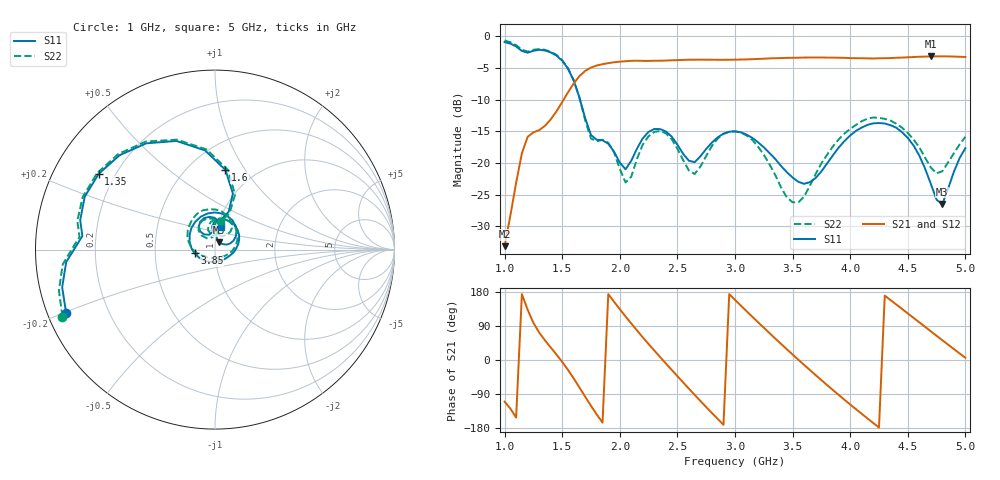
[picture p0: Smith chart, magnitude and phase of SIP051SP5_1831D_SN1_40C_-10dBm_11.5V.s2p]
# GHz  S  dB  R  50
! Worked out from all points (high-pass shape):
!   81 points, 1 GHz to 5 GHz, reference 50 ohm
!   highest |S21| = -3.16 dB at 4.7 GHz (marker M1); lowest = -33.1 dB at 1 GHz (marker M2)
!   |S21| within 3 dB of the highest: 1.656 GHz to end of sweep
!   lowest |S11| = -26.5 dB at 4.8 GHz (marker M3), VSWR 1.10, Z = 52.1 + j4.36 ohm
!   |S11| at or under -10 dB: 1.655 GHz to end of sweep
!   |S22| runs from -26.2 to -0.6 dB; largest |S21 - S12| = 0.0019
!   S11 on the Smith chart (normalised r, x): 1 GHz: 0.05, -0.20; 1.35 GHz: 0.14, +0.29; 1.6 GHz: 0.74, +0.82; 3.85 GHz: 0.80, -0.03; 5 GHz: 1.04, +0.27
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1  -0.90 -157.0  -33.14 -110.0  -33.15 -110.7  -0.65 -156.3
1.15  -2.31 177.6  -18.47 173.9  -18.47 173.6  -2.10 178.3
1.35  -2.23 146.9  -14.13 51.9  -14.16 52.0  -2.12 147.1
1.5  -3.84 109.6  -10.37 -5.1  -10.35 -5.0  -3.77 109.1
1.6  -6.99 82.5  -7.43 -48.7  -7.42 -48.7  -6.94 80.8
1.7  -12.96 70.1  -5.44 -97.2  -5.45 -97.3  -13.28 68.2
1.9  -16.96 91.7  -4.23 173.8  -4.24 173.9  -16.81 90.1
2.1  -19.63 125.9  -3.86 96.1  -3.87 96.0  -22.14 125.8
2.35  -14.65 99.6  -3.85 7.7  -3.85 7.7  -14.96 103.4
2.5  -17.10 78.4  -3.76 -42.6  -3.76 -42.6  -17.75 77.7
2.65  -19.87 90.7  -3.69 -92.0  -3.69 -92.0  -21.74 94.2
2.85  -15.94 87.0  -3.70 -155.6  -3.71 -155.6  -16.15 98.7
3  -15.00 60.9  -3.68 158.7  -3.67 158.7  -15.03 68.6
3.3  -18.44 4.1  -3.48 70.9  -3.48 70.8  -20.22 -3.3
3.5  -22.30 -40.4  -3.38 14.5  -3.39 14.4  -26.21 -78.9
3.7  -22.37 -115.6  -3.34 -39.9  -3.35 -39.9  -21.73 -156.2
3.85  -18.79 -169.4  -3.35 -79.3  -3.36 -79.3  -17.39 173.0
4.1  -14.40 124.6  -3.46 -142.0  -3.45 -142.1  -13.40 124.8
4.35  -14.03 69.5  -3.43 158.2  -3.44 158.2  -13.30 80.5
4.7  -23.31 23.8  -3.16 75.7  -3.17 75.7  -20.72 57.1
4.8  -26.48 61.7  -3.16 52.1  -3.17 52.1  -21.31 78.2
5  -17.66 74.4  -3.25 5.9  -3.27 5.9  -15.86 78.1
